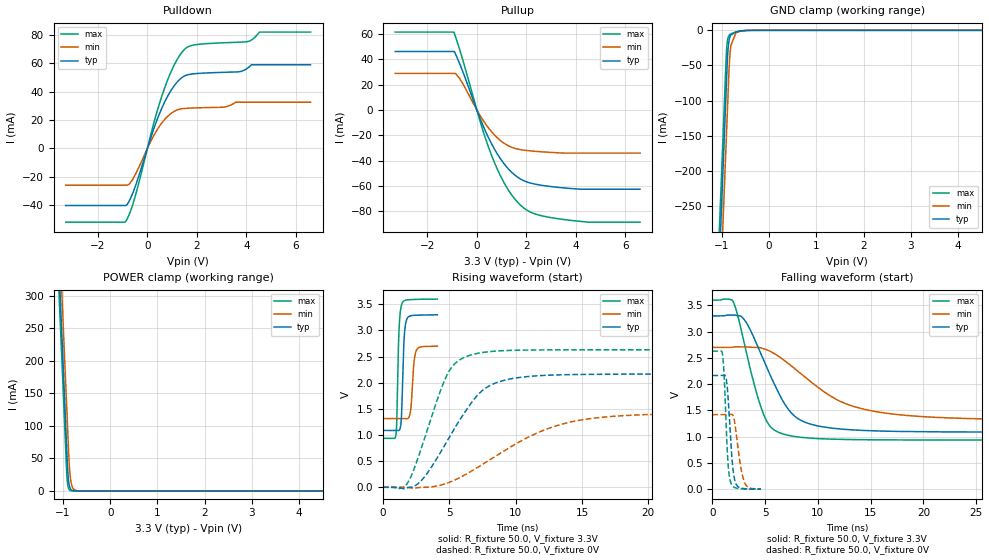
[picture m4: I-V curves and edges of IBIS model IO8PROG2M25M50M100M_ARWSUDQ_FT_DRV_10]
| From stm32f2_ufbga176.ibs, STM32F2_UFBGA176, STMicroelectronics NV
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| *** New cell (Generated with 5.14beta1 (Sep 20 2010 13:23:23))
[Model]   IO8PROG2M25M50M100M_ARWSUDQ_FT_DRV_10
Model_type 3-state
Polarity   Non-Inverting
Enable   Active-Low
| CAP_THRESHOLD on pad IOV33 is "CMOS" :
| Rising=10.0% of vddio   Falling=90.0% of vddio
| C_comp min and max val. don't necessarily correlate with the min and max pvt
| but are the smallest and greatest pad capacitance found.
| var   typ   min   max
C_comp   2.32810pF  2.21810pF  2.46460pF
Vmeas = 1.65V   | Reference voltage for timing measurements
Cref  = 50.0pF   | Timing specification test load capacitance value
Rref  = 10.0MOhm   | Timing specification test load resistance value
Vref  = 1.65V   | Timing specification test load voltage
[Model Spec]
| variable   typ   min   max
[Temperature Range] 25.0 125.0 -40.0
| variable   typ   min   max
[Voltage Range] 3.3V 2.7V 3.6V
| variable   typ   min   max
[POWER Clamp Reference] 3.3V 2.7V 3.6V
| variable   typ   min   max
[GND Clamp Reference] 0V 0V 0V
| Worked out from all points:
|   slope of the pulldown table from 0 to 0.495 V, typ, clamps not added: 20 ohm
|   slope of the pullup table from 0 to 0.495 V, typ, clamps not added: 21.7 ohm
|   GND clamp passes 1 mA (typ) near -0.61 V on its own axis
|   POWER clamp passes 1 mA (typ) near -0.81 V on its own axis
|   rising waveform, R_fixture 50.0, V_fixture 3.3V: 20-80 % time 174ps typ, 218ps min, 160ps max; typ from 1.09 V to 3.3 V
|   falling waveform, R_fixture 50.0, V_fixture 3.3V: 20-80 % time 3.17ns typ, 6.13ns min, 2.08ns max; typ from 3.3 V to 1.09 V
|   rising waveform, R_fixture 50.0, V_fixture 0V: 20-80 % time 3.26ns typ, 6.08ns min, 2.15ns max; typ from 0 V to 2.17 V
|   falling waveform, R_fixture 50.0, V_fixture 0V: 20-80 % time 429ps typ, 610ps min, 343ps max; typ from 2.17 V to 0.001 V
[POWER Clamp]
-3.3V     4.11A      4.173A     4.072A
-1.09V    352.5mA    415.9mA    314.5mA
-1.05V    284.5mA    347.9mA    246.5mA
-1.01V    216.5mA    279.9mA    178.5mA
-920mV    63.51mA    126.9mA    25.85mA
-900mV    31.51mA    92.9mA     9.552mA
-890mV    21.35mA    75.9mA     5.807mA
-870mV    9.804mA    44.01mA    2.146mA
-840mV    3.05mA     18.36mA    482.1uA
-780mV    295.2uA    3.194mA    24.34uA
-660mV    2.764uA    96.52uA    62.42nA
6.6V      0A         0A         0A
[GND Clamp]
-3.3V     -4.149A    -4.224A    -4.103A
-1.06V    -341mA     -415.8mA   -295.1mA
-940mV    -137mA     -211.8mA   -91.11mA
-910mV    -86.01mA   -160.8mA   -40.11mA
-900mV    -69.01mA   -143.8mA   -27.13mA
-880mV    -37.2mA    -109.8mA   -14.07mA
-860mV    -20.02mA   -75.82mA   -8.837mA
-840mV    -11.77mA   -45.3mA    -6.542mA
-810mV    -6.468mA   -21.54mA   -4.94mA
-700mV    -2.247mA   -3.206mA   -2.168mA
-470mV    -130uA     -313.8uA   -60.76uA
6.6V      10.47nA    1.304uA    84.25pA
| variable   typ   min   max
[Pullup Reference] 3.3V 2.7V 3.6V
| variable   typ   min   max
[Pulldown Reference] 0V 0V 0V
[Pullup]
-3.3V     45.98mA    28.79mA    61.32mA
-930mV    45.98mA    28.79mA    61.32mA
-700mV    36.75mA    24.83mA    47.96mA
120mV     -6.142mA   -4.065mA   -8.189mA
590mV     -26.5mA    -17.07mA   -35.52mA
1.18V     -44.36mA   -27.27mA   -60.11mA
1.54V     -51.43mA   -30.39mA   -70.35mA
1.89V     -55.75mA   -31.69mA   -77.18mA
2.48V     -58.98mA   -32.83mA   -82.75mA
3.6V      -61.62mA   -34.07mA   -86.61mA
4.51V     -62.54mA   -34.07mA   -88.51mA
6.6V      -62.54mA   -34.07mA   -88.51mA
[Pulldown]
-3.3V     -40.26mA   -25.94mA   -51.99mA
-870mV    -40.25mA   -25.94mA   -51.33mA
-720mV    -36.35mA   -24.93mA   -45.5mA
-470mV    -25.89mA   -17.87mA   -32.39mA
240mV     12.97mA    8.52mA     16.62mA
590mV     28.62mA    18.11mA    37.2mA
1.07V     43.85mA    26mA       58.31mA
1.54V     51.42mA    28.24mA    70.48mA
2.01V     52.82mA    28.63mA    73.27mA
4.01V     56.05mA    32.64mA    75.18mA
4.53V     59mA       32.64mA    82.02mA
6.6V      59mA       32.64mA    82.02mA
[Ramp]
dV/dt_r 1.29886V/3.25662ns 851.30596mV/6.08237ns 1.57728V/2.15392ns
dV/dt_f 1.32782V/3.1672ns 831.60153mV/6.13969ns 1.59819V/2.07784ns
R_load = 50.0
| Removed startup time: 0s 0s 0s  .
| Removed end time: 4.098ns.
[Rising Waveform]
R_fixture   = 50.0
V_fixture   = 3.3V
V_fixture_min = 2.7V
V_fixture_max = 3.6V
0s        1.087V     1.314V     936.3mV
979ps     1.087V     1.314V     1.004V
1.042ns   1.086V     1.314V     1.283V
1.206ns   1.086V     1.314V     2.988V
1.421ns   1.526V     1.314V     3.506V
1.584ns   2.808V     1.313V     3.563V
1.793ns   3.21V      1.309V     3.581V
2.084ns   3.279V     1.469V     3.588V
2.5ns     3.29V      2.608V     3.593V
4.1ns     3.298V     2.697V     3.598V
| Removed startup time: 0s 0s 0s  .
| Removed end time: 44.05ns.
[Falling Waveform]
R_fixture   = 50.0
V_fixture   = 3.3V
V_fixture_min = 2.7V
V_fixture_max = 3.6V
0s        3.3V       2.7V       3.6V
1.95ns    3.316V     2.706V     3.578V
3.115ns   3.202V     2.71V      2.69V
4.755ns   2.503V     2.681V     1.475V
5.48ns    2.17V      2.624V     1.193V
6.69ns    1.677V     2.47V      1.051V
9.255ns   1.242V     2.056V     972.6mV
12.37ns   1.142V     1.65V      947.8mV
16.02ns   1.107V     1.46V      939.6mV
44.06ns   1.087V     1.315V     936.3mV
| Removed startup time: 0s 0s 0s  .
| Removed end time: 34.51ns.
[Rising Waveform]
R_fixture   = 50.0
V_fixture   = 0V
V_fixture_min = 0V
V_fixture_max = 0V
0s        8.028nV    322.2nV    5.736nV
1.87ns    -7.114mV   -2.513mV   87.92mV
2.995ns   156.4mV    -2.011mV   827mV
4.805ns   870.9mV    75.77mV    2.134V
6.54ns    1.573V     289.5mV    2.523V
7.595ns   1.871V     451.8mV    2.58V
9.105ns   2.043V     691.4mV    2.612V
12.3ns    2.14V      1.109V     2.626V
15.39ns   2.158V     1.305V     2.628V
34.52ns   2.165V     1.419V     2.629V
| Removed startup time: 0s 0s 0s  .
| Removed end time: 4.592ns.
[Falling Waveform]
R_fixture   = 50.0
V_fixture   = 0V
V_fixture_min = 0V
V_fixture_max = 0V
0s        2.165V     1.419V     2.629V
961ps     2.166V     1.419V     2.558V
1.144ns   2.171V     1.419V     2.028V
1.358ns   2.03V      1.418V     937.7mV
1.525ns   1.62V      1.42V      375.4mV
1.735ns   904.3mV    1.426V     127.3mV
1.98ns    325.8mV    1.389V     46.81mV
2.283ns   81.96mV    1.014V     19.88mV
3.071ns   10.08mV    115.6mV    3.431mV
4.594ns   1.296mV    3.006mV    725.1uV
